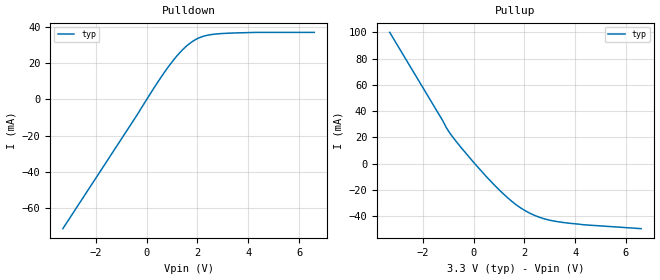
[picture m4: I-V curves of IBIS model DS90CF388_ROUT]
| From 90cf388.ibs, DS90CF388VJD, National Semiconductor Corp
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|   RECEIVER Output  MODEL
[Model]   DS90CF388_ROUT
Model_type   Output
| Signals   Rs,Gs & Bs
Vmeas = 1.5V
Cref = 8pF   |Timing specification test load capacitance value
Rref = 1000.0
Vref = 0.0   |Timing specification test load voltage; GND
Vinl = 0.8
Vinh = 2.0
| variable   typ   min   max
C_comp   5.753pF   NA   NA
|   typ   min   max
[Temperature Range]   25.0   -10   70
[Voltage range]   3.3V   3.0V   3.6V
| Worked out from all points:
|   slope of the pulldown table from 0 to 0.495 V, typ, clamps not added: 45.8 ohm
|   slope of the pullup table from 0 to 0.495 V, typ, clamps not added: 46 ohm
[Pulldown]
| Voltage   I(typ)   I(min)   I(max)
-3.3V     -71.3mA    NA         NA
-399mV    -9.013mA   NA         NA
582mV     12.6mA     NA         NA
1.194V    24.08mA    NA         NA
1.439V    27.78mA    NA         NA
1.685V    30.8mA     NA         NA
1.93V     33.07mA    NA         NA
2.174V    34.6mA     NA         NA
2.787V    36.18mA    NA         NA
4.256V    37mA       NA         NA
6.6V      37mA       NA         NA
[Pullup]
| Note that the[Pullup]voltage table is referenced to Vcc
| and is calculated using Vtable=Vcc - Vmeasured.
|Voltage   I(typ)   I(min)   I(max)
-3.3V     100mA      NA         NA
-1.202V   32.39mA    NA         NA
-1.08V    27.74mA    NA         NA
-835mV    20.71mA    NA         NA
-470mV    11.79mA    NA         NA
513mV     -10.02mA   NA         NA
1.125V    -22.1mA    NA         NA
1.615V    -30.38mA   NA         NA
2.352V    -38.93mA   NA         NA
3.083V    -43.39mA   NA         NA
4.311V    -46.49mA   NA         NA
6.6V      -49.49mA   NA         NA
[GND_clamp]
| Outputs in Tri-state.
| Voltage   I(typ)   I(min)   I(max)
-3.3V     0A         0A         0A
3V        0A         0A         0A
[POWER_clamp]
| Note that the[POWER_clamp]voltage table is referenced to Vcc
| and is calculated using Vtable=Vcc - Vmeasured.
| Outputs in Tri-state.
|Voltage   I(typ)   I(min)   I(max)
-3.3V     0A         0A         0A
3.3V      0A         0A         0A
[Ramp]
|   typ   min   max
dV/dt_r   1.865/1.98n   NA   NA
dV/dt_f   1.865/2.25n   NA   NA
R_load = 1000Ohm
